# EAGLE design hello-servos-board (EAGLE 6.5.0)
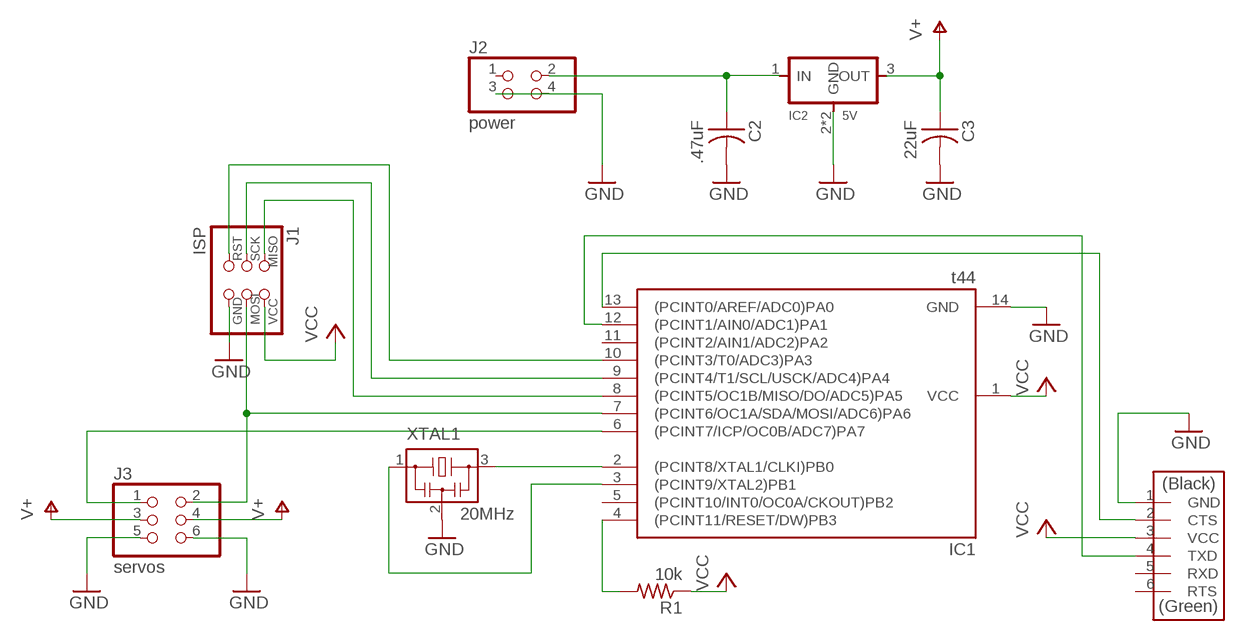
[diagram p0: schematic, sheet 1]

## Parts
C2  .47uF  CAP-US1206FAB  [C1206FAB]
C3  22uF  CAP-US1206FAB  [C1206FAB]
FTDI  FTDI-SMD-HEADER  [1X06SMD]
IC1  t44  ATTINY44-SSU  [SOIC14]
IC2  5V  REGULATORSOT223  [SOT223]
J1  ISP  AVRISPSMD  [2X03SMD]
J2  power  PINHD-2X2-SMD  [2X02SMD]
J3  servos  PINHD-2X3-SMD  [2X03SMD]
R1  10k  RES-US1206FAB  [R1206FAB]
XTAL1  20MHz  RESONATOR  [EFOBM]

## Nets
GND: C2.2 C3.2 FTDI.1(GND) IC1.14(GND) IC2.2(GND) IC2.4(GND) J1.6(GND) J2.3 J2.4 J3.5 J3.6 XTAL1.2
N$1: IC1.2((PCINT8/XTAL1/CLKI)PB0) XTAL1.3
N$2: IC1.3((PCINT9/XTAL2)PB1) XTAL1.1
N$3: IC1.6((PCINT7/ICP/OC0B/ADC7)PA7) J3.1
N$4: IC1.7((PCINT6/OC1A/SDA/MOSI/ADC6)PA6) J1.4(MOSI) J3.2
N$5: IC1.4((PCINT11/RESET/DW)PB3) R1.2
N$6: IC1.8((PCINT5/OC1B/MISO/DO/ADC5)PA5) J1.1(MISO)
N$7: IC1.9((PCINT4/T1/SCL/USCK/ADC4)PA4) J1.3(SCK)
N$8: IC1.10((PCINT3/T0/ADC3)PA3) J1.5(RST)
N$9: C2.1 IC2.1(IN) J2.2
N$10: FTDI.4(TXD) IC1.12((PCINT1/AIN0/ADC1)PA1)
N$12: FTDI.2(CTS) IC1.13((PCINT0/AREF/ADC0)PA0)
V+: C3.1 IC2.3(OUT) J3.3 J3.4
VCC: FTDI.3(VCC) IC1.1(VCC) J1.2(VCC) R1.1
Unconnected: FTDI.5(RXD) FTDI.6(RTS) IC1.5((PCINT10/INT0/OC0A/CKOUT)PB2) IC1.11((PCINT2/AIN1/ADC2)PA2) J2.1

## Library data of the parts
C2 C3 = fab:CAP-US
FTDI = fab:FTDI-SMD-HEADER
IC1 = fab:ATTINY44
IC2 = fab:REGULATOR
J1 = fab:AVRISP
J2 = fab:PINHD-2X2-SMD
J3 = fab:PINHD-2X3-SMD: PIN HEADER
R1 = fab:RES-US: Resistor (US Symbol)
XTAL1 = fab:RESONATOR

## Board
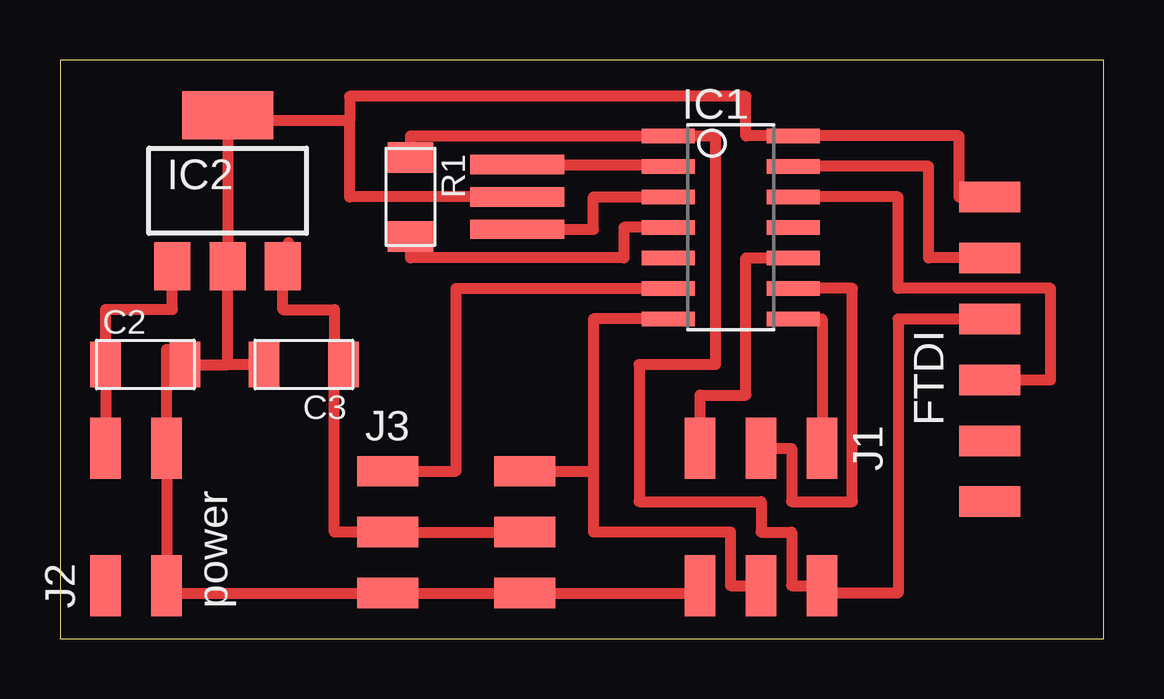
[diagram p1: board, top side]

Size 43.48 x 24.12 mm. Coordinates in mm from the lower left corner, seen from the top.
Outline: 0,0 43.48,0 43.48,24.12 0,24.12 0,0
Copper layers (1*16): Top 0.035mm / dielectric 1.5mm / Bottom 0.035mm
Design rules "design-rules-fablab": minimum track width 18mil, minimum drill 24mil, track to track 0.4mm, track to pad 0.4mm, pad to pad 0.4mm, via to via 0.4mm, smd to smd 8mil, copper to edge 1mil, drill to drill 8mil, minimum pad ring 10mil, minimum via ring 8mil, stop-mask expansion 4mil, vias tented up to drill 0mil, thermal gap 10mil

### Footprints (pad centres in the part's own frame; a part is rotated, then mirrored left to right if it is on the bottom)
C1206FAB = smd 1.27 x 1.905: 1 -1.651,0; 2 1.651,0
1X06SMD = smd 2.54 x 1.27: 1 0,6.35; 2 0,3.81; 3 0,1.27; 4 0,-1.27; 5 0,-3.81; 6 0,-6.35
SOIC14 = smd 0.61 x 2.21: 1 -3.81,-2.603; 2 -2.54,-2.603; 3 -1.27,-2.603; 4 0,-2.603; 5 1.27,-2.603; 6 2.54,-2.603; 7 3.81,-2.603; 8 3.81,2.603; 9 2.54,2.603; 10 1.27,2.603; 11 0,2.603; 12 -1.27,2.603; 13 -2.54,2.603; 14 -3.81,2.603
SOT223 = smd 1.5 x 2: 1 -2.3,-3.15; 2 0,-3.15; 3 2.3,-3.15 | smd 3.8 x 2: 4 0,3.15
2X03SMD = smd 2.54 x 1.27: 1 -2.857,2.54; 2 2.857,2.54; 3 -2.857,0; 4 2.857,0; 5 -2.857,-2.54; 6 2.857,-2.54
2X02SMD = smd 2.54 x 1.27: 1 -2.857,1.27; 2 2.857,1.27; 3 -2.857,-1.27; 4 2.857,-1.27
R1206FAB = smd 1.27 x 1.905: 1 -1.651,0; 2 1.651,0
EFOBM = smd 0.8 x 3.9: 1 -1.35,0; 2 0,0; 3 1.35,0

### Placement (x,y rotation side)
C2  3.56,11.43 0 top
C3  10.16,11.43 180 top
FTDI  38.73,12.06 0 top
IC1  27.94,17.14 270 top
IC2  6.99,18.67 0 top
J1  29.21,5.08 270 top
J2  3.17,5.08 90 top
J3  16.51,4.45 0 top
R1  14.61,18.41 270 top
XTAL1  19.05,18.41 90 top

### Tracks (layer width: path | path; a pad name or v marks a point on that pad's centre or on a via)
GND
  Top 0.457: J1.6 26.67,1.91 J3.6 J3.5 4.45,1.91 J2.3 J2.4 4.45,12.06 5.08,12.06 5.08,11.43 C2.2 6.99,11.43 | C3.2 6.99,11.43 | 6.99,11.43 IC2.2 6.99,21.59 | XTAL1.2 12.06,18.41 12.06,21.59 | 12.06,21.59 6.99,21.59 | IC2.4 6.99,21.59 | FTDI.1 37.47,18.41 37.47,20.95 IC1.14 28.57,20.95 28.57,22.61 12.06,22.61 12.06,21.59
N$1
  Top 0.457: XTAL1.3 25.34,19.77 IC1.2
N$2
  Top 0.457: XTAL1.1 22.23,17.07 22.23,18.41 IC1.3
N$3
  Top 0.457: J3.1 16.51,6.99 16.51,14.61 IC1.6
N$4
  Top 0.457: IC1.7 22.23,13.34 22.23,6.99 | 22.23,6.99 22.23,4.45 27.94,4.45 27.94,2.22 J1.4 | J3.2 22.23,6.99
N$5
  Top 0.457: IC1.4 23.5,17.14 23.5,15.88 14.61,15.88 R1.2
N$6
  Top 0.457: IC1.8 31.75,13.34 J1.1
N$7
  Top 0.457: IC1.9 33.02,14.61 33.02,5.71 30.48,5.71 30.48,7.94 J1.3
N$8
  Top 0.457: J1.5 26.67,10.16 28.57,10.16 28.57,15.88 IC1.10
N$9
  Top 0.457: IC2.1 4.68,13.72 1.91,13.72 C2.1 J2.2
N$10
  Top 0.457: FTDI.4 41.27,10.79 41.27,14.61 34.92,14.61 34.92,18.41 IC1.12
N$12
  Top 0.457: FTDI.2 36.2,15.88 36.2,19.68 IC1.13
V+
  Top 0.457: J3.4 J3.3 11.43,4.45 11.43,11.43 | 9.53,16.51 9.53,15.9 IC2.3 9.29,13.72 11.43,13.72 11.43,11.43 | C3.1 11.43,11.43
VCC
  Top 0.457: FTDI.3 34.92,13.34 34.92,1.91 31.75,1.91 J1.2 30.48,2.22 30.48,4.45 29.21,4.45 29.21,5.71 24.13,5.71 24.13,11.43 27.3,11.43 27.3,20.95 IC1.1 14.61,20.95 R1.1 15.24,20.07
